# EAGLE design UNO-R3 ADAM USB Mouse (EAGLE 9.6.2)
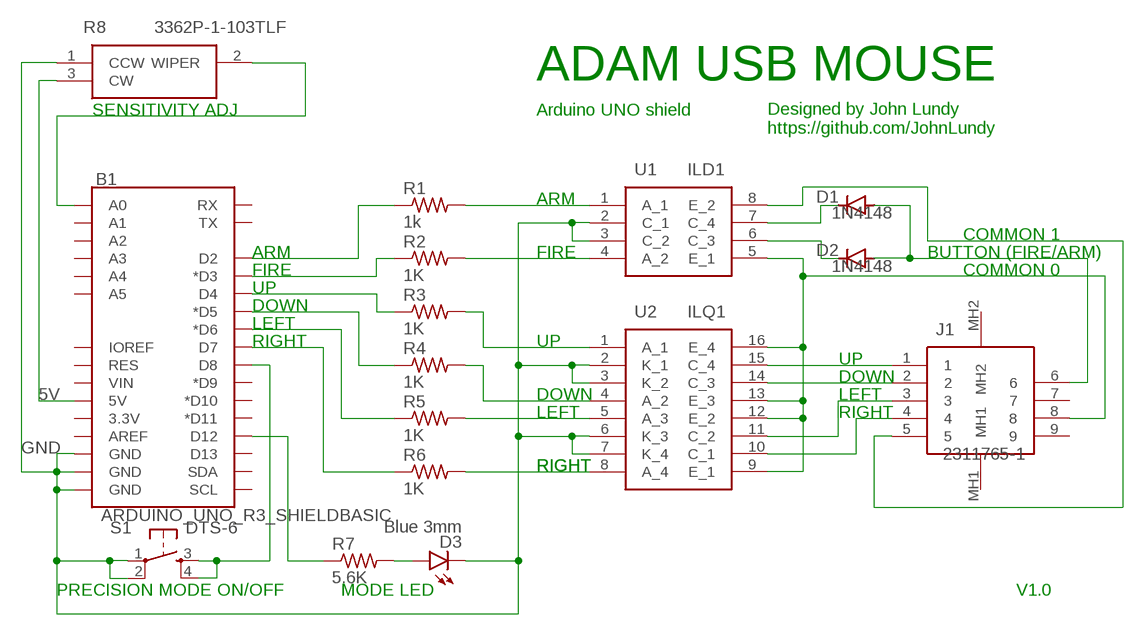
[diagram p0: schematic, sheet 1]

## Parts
B1  ARDUINO_UNO_R3_SHIELDBASIC  [UNO_R3_SHIELD]
D1  1N4148  1N4148DO35-7  [DO35-7]
D2  1N4148  1N4148DO35-7  [DO35-7]
D3  Blue 3mm  LED3MM  [LED3MM]
J1  2311765-1  [23117651]
R1  1k  R-US_0204/7  [0204/7]
R2  1K  R-US_0204/7  [0204/7]
R3  1K  R-US_0204/7  [0204/7]
R4  1K  R-US_0204/7  [0204/7]
R5  1K  R-US_0204/7  [0204/7]
R6  1K  R-US_0204/7  [0204/7]
R7  5.6K  R-US_0204/7  [0204/7]
R8  3362P-1-103TLF  [3296P-1-103]
S1  DTS-6  [DTS-6]
U1  ILD1  ILD2  [DIP762W56P254L977H470Q8N]
U2  ILQ1  [DIP762W56P254L1992H470Q16N]

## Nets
5V [Supply]: B1.5V R8.3(CW)
GND [Supply]: B1.GND@0(GND) B1.GND@1(GND) B1.GND@2(GND) D3.K(C) R8.1(CCW) S1.1 S1.2 U1.2(C_1) U1.3(C_2) U2.2(K_1) U2.3(K_2) U2.6(K_3) U2.7(K_4)
N$1: B1.D2 R1.1
N$2: B1.D3(*D3) R2.1
N$3: B1.D4 R3.1
N$4: B1.D5(*D5) R4.1
N$5: B1.D6(*D6) R5.1
N$6: B1.D7 R6.1
N$7: R1.2 U1.1(A_1)
N$8: R2.2 U1.4(A_2)
N$9: R3.2 U2.1(A_1)
N$10: R4.2 U2.4(A_2)
N$11: R5.2 U2.5(A_3)
N$12: R6.2 U2.8(A_4)
N$13: D1.C U1.7(C_4)
N$14: D2.C U1.6(C_3)
N$15: J1.5 U1.8(E_2)
N$17: J1.1 U2.15(C_4)
N$18: J1.8 U1.5(E_1) U2.9(E_1) U2.12(E_2) U2.13(E_3) U2.16(E_4)
N$20: B1.A0 R8.2(WIPER)
N$21: B1.D8 S1.3 S1.4
N$22: B1.D12 R7.1
N$23: D3.A R7.2
N$24: J1.2 U2.14(C_3)
N$25: D1.A D2.A J1.6
N$26: J1.3 U2.11(C_2)
N$27: J1.4 U2.10(C_1)
Unconnected: B1.3.3V B1.A1 B1.A2 B1.A3 B1.A4 B1.A5 B1.AREF B1.D9(*D9) B1.D10(*D10) B1.D11(*D11) B1.D13 B1.IOREF B1.RES B1.RX B1.SCL B1.SDA B1.TX B1.VIN J1.7 J1.9 J1.MH1 J1.MH2

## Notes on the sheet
- ADAM USB MOUSE
- SENSITIVITY ADJ | Arduino UNO shield
- Designed by John Lundy
  https://github.com/JohnLundy
- ARM
- COMMON 1
- ARM | FIRE | BUTTON (FIRE/ARM)
- FIRE | COMMON 0
- UP
- DOWN
- LEFT
- RIGHT | UP
- UP
- DOWN
- DOWN | LEFT
- LEFT | RIGHT
- RIGHT | RIGHT
- PRECISION MODE ON/OFF | MODE LED | V1.0

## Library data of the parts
B1 = SparkFun-Boards:ARDUINO_UNO_R3_SHIELD: Arduino R3 Shield Footprint Shield form compatible with the Arduino Uno R3. SparkFun Products: MG2639 Cellular Shield MIDI Shield R3 Stackable Headers Kit
D1 D2 = diode:1N4148: DIODE
D3 = led:LED: LED
J1 = SamacSys_Parts:2311765-1: AMPLIMITE HD22 Board Mount Connectors: AMPL REC, HD20, R/A, 9P, S/L, .318 Source: Datasheet; ARROW_PART_NUMBER: 2311765-1; ARROW_PRICE-STOCK: https://www.arrow.com/en/products/2311765-1/te-connectivity; DESCRIPTION: AMPLIMITE HD22 Board Mount Connectors: AMPL REC, HD20, R/A, 9P, S/L, .318; HEIGHT: 12.8mm; MANUFACTURER_NAME: TE Connectivity; MANUFACTURER_PART_NUMBER: 2311765-1; MOUSER_PART_NUMBER: 571-2311765-1; MOUSER_PRICE-STOCK: https://www.mouser.co.uk/ProductDetail/TE-Connectivity/2311765-1?qs=rrS6PyfT74ebQi5fQFugmA%3D%3D
R1-R7 = adafruit:R-US_: RESISTOR, American symbol
R8 = SamacSys_Parts:3362P-1-103TLF: BOURNS - 3362P-1-103TLF - TRIMMER POTENTIOMETER, 10KOHM 1TURN THROUGH HOLE Source: Datasheet; ARROW_PART_NUMBER: 3362P-1-103TLF; ARROW_PRICE-STOCK: https://www.arrow.com/en/products/3362p-1-103tlf/bourns; DESCRIPTION: BOURNS - 3362P-1-103TLF - TRIMMER POTENTIOMETER, 10KOHM 1TURN THROUGH HOLE; HEIGHT: mm; MANUFACTURER_NAME: Bourns; MANUFACTURER_PART_NUMBER: 3362P-1-103TLF; MOUSER_PART_NUMBER: 652-3362P-1-103TLF; MOUSER_PRICE-STOCK: https://www.mouser.co.uk/ProductDetail/Bourns/3362P-1-103TLF?qs=izR6mho4f8VBTlFqy0U7Gg%3D%3D
S1 = switch-tact:DTS-6
U1 = SamacSys_Parts:ILD2: Transistor Output Optocouplers Phototransistor Out Dual CTR >100% Source: Datasheet; ARROW_PART_NUMBER: ILD2; ARROW_PRICE-STOCK: https://www.arrow.com/en/products/ild2/vishay; DESCRIPTION: Transistor Output Optocouplers Phototransistor Out Dual CTR >100%; HEIGHT: 4.7mm; MANUFACTURER_NAME: Vishay; MANUFACTURER_PART_NUMBER: ILD2; MOUSER_PART_NUMBER: 782-ILD2; MOUSER_PRICE-STOCK: https://www.mouser.co.uk/ProductDetail/Vishay-Semiconductors/ILD2/?qs=xCMk%252BIHWTZN1gQU5Qacjxw%3D%3D
U2 = SamacSys_Parts:ILQ1: Optocoupler DC-IN 4-CH Trans DC-OUT Source: Datasheet; ARROW_PART_NUMBER: ILQ1; ARROW_PRICE-STOCK: https://www.arrow.com/en/products/ilq1/vishay; DESCRIPTION: Optocoupler DC-IN 4-CH Trans DC-OUT; HEIGHT: 4.7mm; MANUFACTURER_NAME: Vishay; MANUFACTURER_PART_NUMBER: ILQ1; MOUSER_PART_NUMBER: 782-ILQ1; MOUSER_PRICE-STOCK: https://www.mouser.co.uk/ProductDetail/Vishay-Semiconductors/ILQ1?qs=MZ2FkKEZZL8rYKp%252BhEUQuQ%3D%3D

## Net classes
0 default: width 0.3 mm
1 Supply: width 0.5 mm

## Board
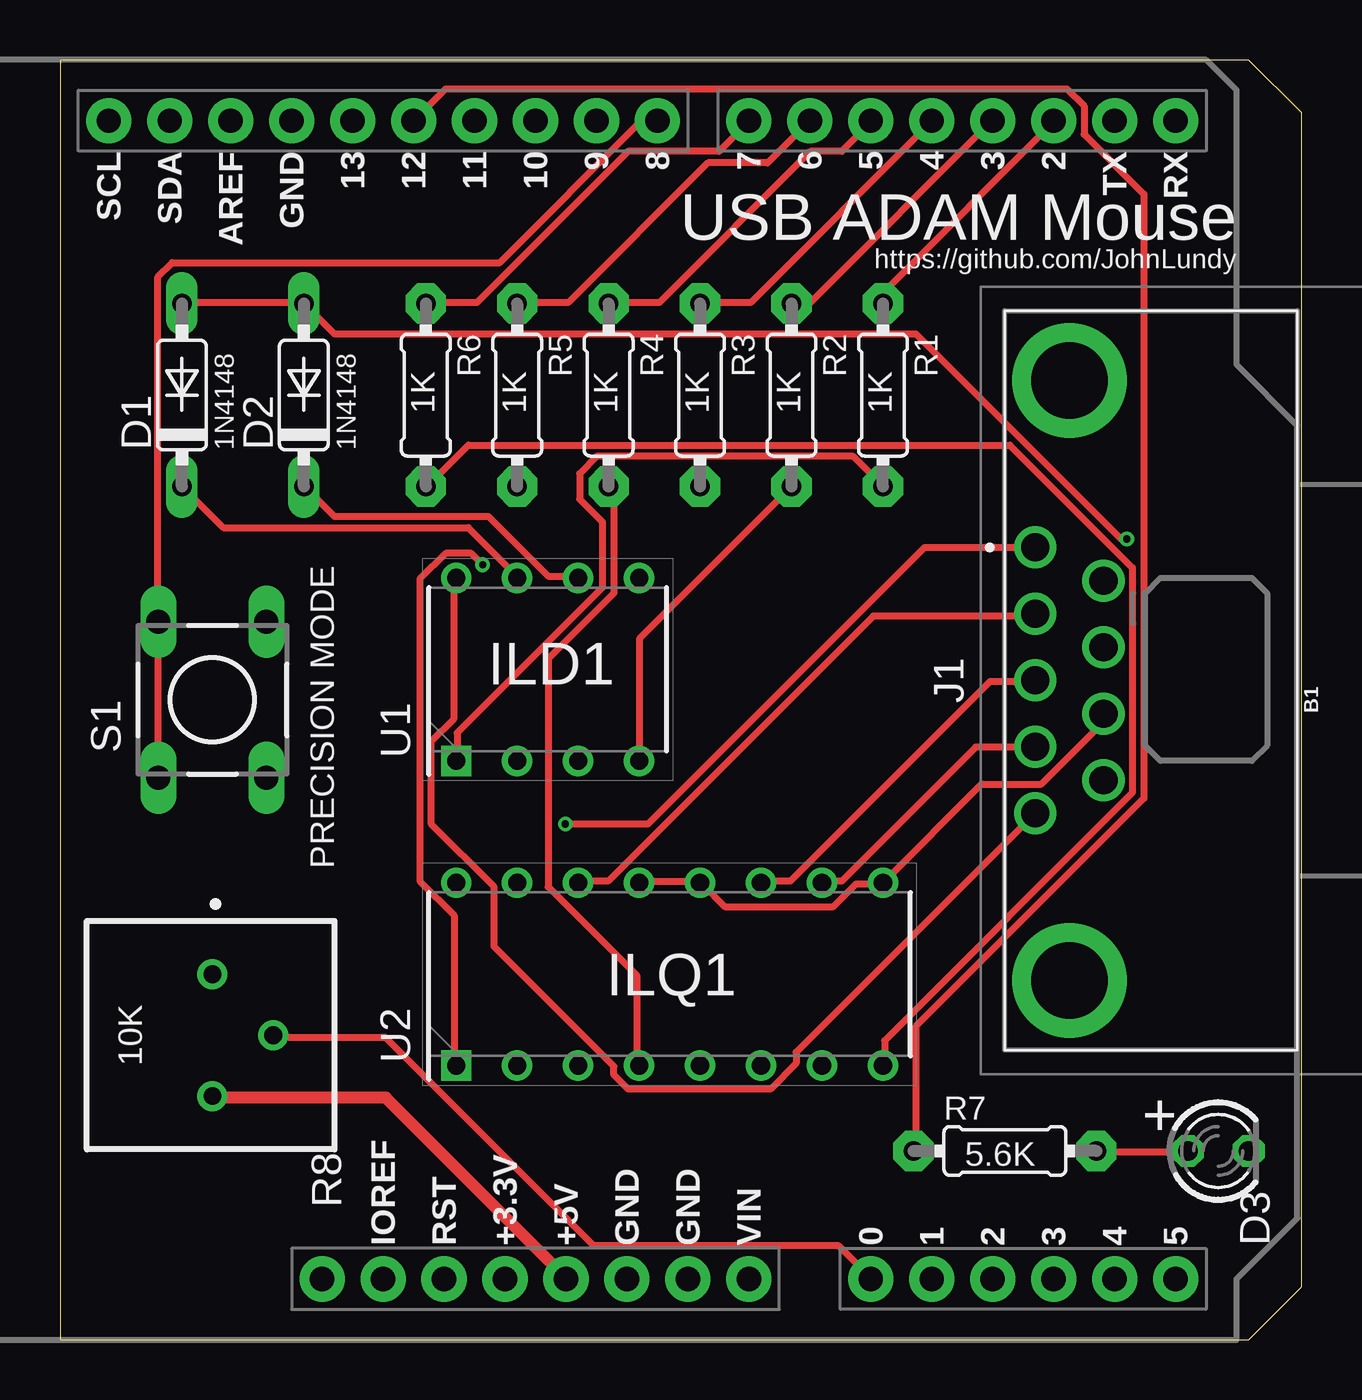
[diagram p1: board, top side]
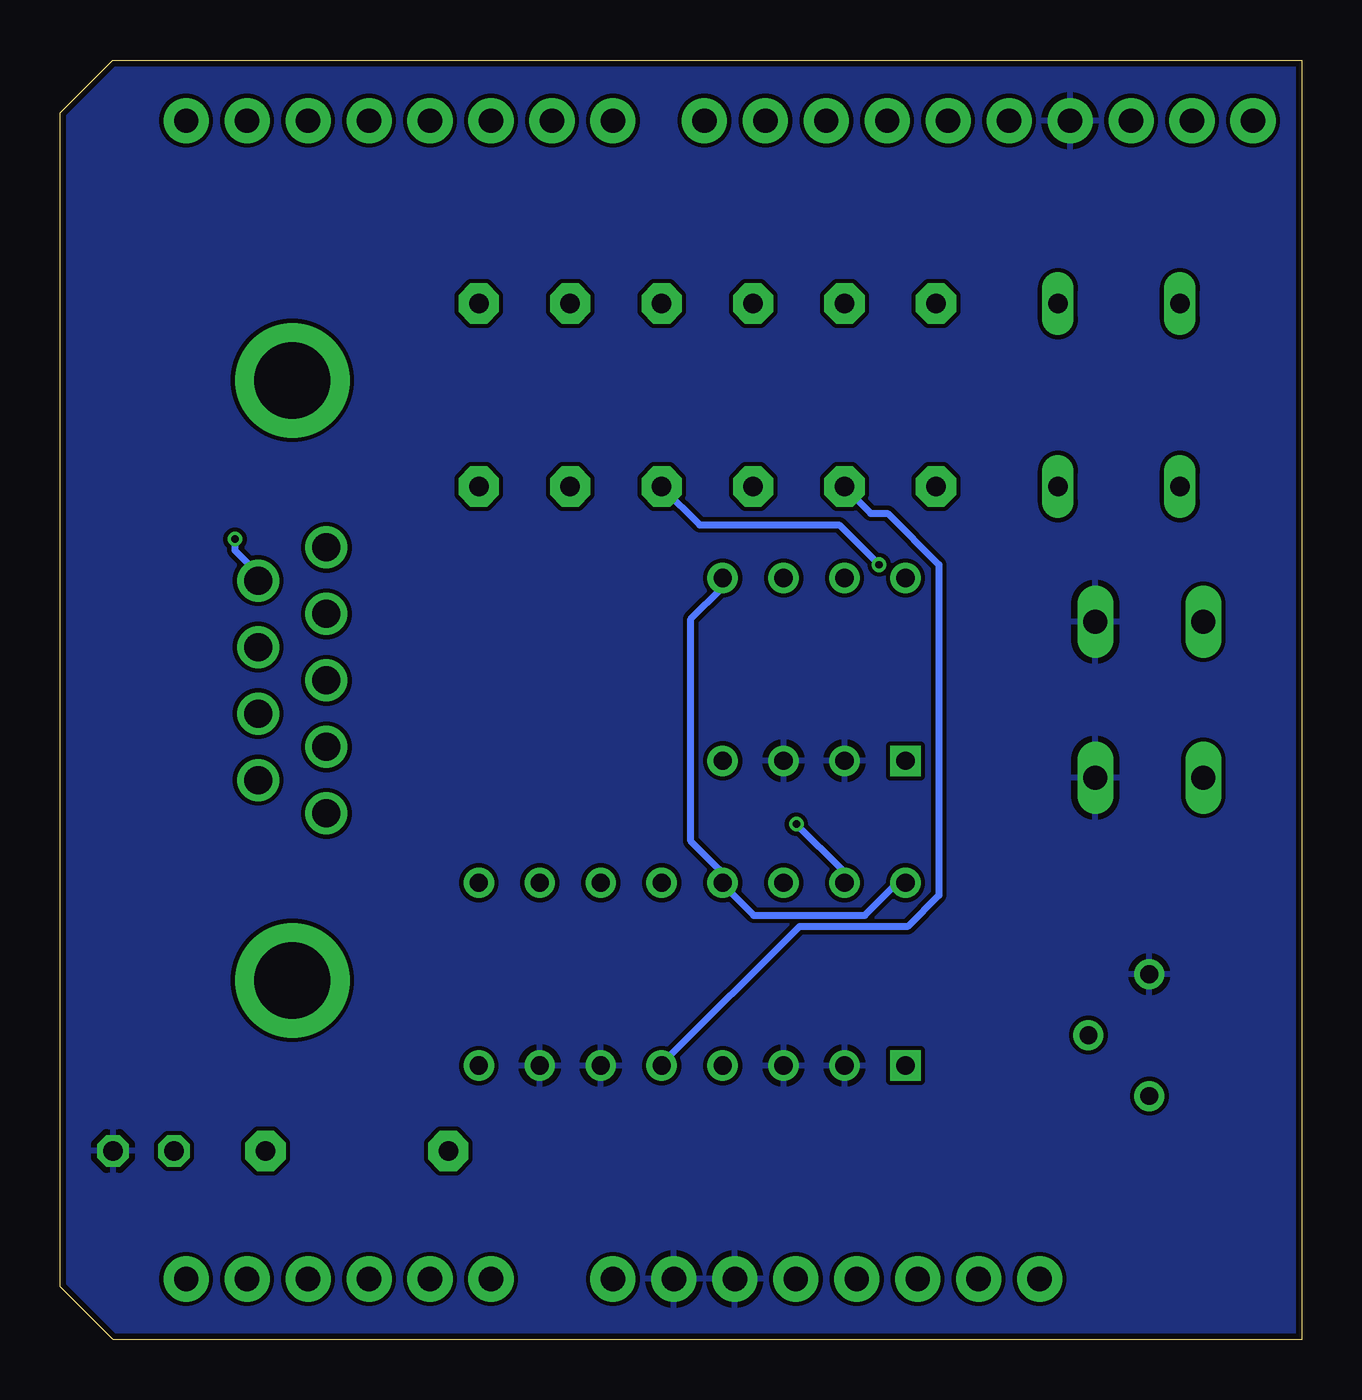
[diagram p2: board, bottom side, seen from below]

Size 51.74 x 53.33 mm. Coordinates in mm from the lower left corner, seen from the top.
Outline: 0,0 49.53,0 51.74,2.21 51.74,51.13 49.54,53.33 0,53.33 0,0
Copper layers (1*16): Top 0.035mm / dielectric 1.5mm / Bottom 0.035mm
Design rules "dirt_cheap_dirty_boards.v1.1 *": minimum track width 6mil, minimum drill 12mil, track to track 0.175mm, track to pad 0.175mm, pad to pad 0.175mm, via to via 6mil, smd to smd 0mil, copper to edge 10mil, drill to drill 10mil, minimum pad ring 10mil, minimum via ring 6mil, stop-mask expansion 2mil, vias tented up to drill 25mil, thermal gap 10mil

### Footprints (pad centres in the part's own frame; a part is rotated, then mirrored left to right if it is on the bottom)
UNO_R3_SHIELD = drill 1.016 pad 1.88: 3.3V 24.13,-2.54; 5V 24.13,0; A0 24.13,12.7; A1 24.13,15.24; A2 24.13,17.78; A3 24.13,20.32; A4 24.13,22.86; A5 24.13,25.4; AREF -24.13,-13.97; D2 -24.13,20.32; D3 -24.13,17.78; D4 -24.13,15.24; D5 -24.13,12.7; D6 -24.13,10.16; D7 -24.13,7.62; D8 -24.13,3.81; D9 -24.13,1.27; D10 -24.13,-1.27; D11 -24.13,-3.81; D12 -24.13,-6.35; D13 -24.13,-8.89; GND@0 24.13,2.54; GND@1 24.13,5.08; GND@2 -24.13,-11.43; IOREF 24.13,-7.62; NC 24.13,-10.16; RES 24.13,-5.08; RX -24.13,25.4; SCL -24.13,-19.05; SDA -24.13,-16.51; TX -24.13,22.86; VIN 24.13,7.62
DO35-7 = drill 0.813 long: A 3.81,0; C -3.81,0
LED3MM = drill 0.813 octagon: A -1.27,0; K 1.27,0
23117651 = drill 1.17 pad 1.755: 1 0,0; 2 -2.77,0; 3 -5.54,0; 4 -8.31,0; 5 -11.08,0; 6 -1.385,-2.84; 7 -4.155,-2.84; 8 -6.925,-2.84; 9 -9.695,-2.84 | drill 3.18 pad 4.77: MH1 -18.04,-1.42; MH2 6.96,-1.42
0204/7 = drill 0.813 pad 1.676 octagon: 1 -3.81,0; 2 3.81,0
3296P-1-103 = drill 0.74 pad 1.24: 1 -2.54,-2.54; 2 0,0; 3 2.54,-2.54
DTS-6 = drill 1 long: 1 -3.25,2.25; 2 3.25,2.25; 3 -3.25,-2.25; 4 3.25,-2.25
DIP762W56P254L977H470Q8N = drill 0.76 pad 1.16 square: 1 -3.81,3.81 | drill 0.76 pad 1.16: 2 -3.81,1.27; 3 -3.81,-1.27; 4 -3.81,-3.81; 5 3.81,-3.81; 6 3.81,-1.27; 7 3.81,1.27; 8 3.81,3.81
DIP762W56P254L1992H470Q16N = drill 0.76 pad 1.16 square: 1 -3.81,8.89 | drill 0.76 pad 1.16: 2 -3.81,6.35; 3 -3.81,3.81; 4 -3.81,1.27; 5 -3.81,-1.27; 6 -3.81,-3.81; 7 -3.81,-6.35; 8 -3.81,-8.89; 9 3.81,-8.89; 10 3.81,-6.35; 11 3.81,-3.81; 12 3.81,-1.27; 13 3.81,1.27; 14 3.81,3.81; 15 3.81,6.35; 16 3.81,8.89

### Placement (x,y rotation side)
B1  21.08,26.67 270 top
D1  5.08,39.37 90 top
D2  10.16,39.37 90 top
D3  48.26,7.87 0 top
J1  40.64,33.02 90 top
R1  34.29,39.37 270 top
R2  30.48,39.37 270 top
R3  26.67,39.37 270 top
R4  22.86,39.37 270 top
R5  19.05,39.37 270 top
R6  15.24,39.37 270 top
R7  39.37,7.87 0 top
R8  8.89,12.7 270 top
S1  6.35,26.67 270 top
U1  20.32,27.94 90 top
U2  25.4,15.24 90 top

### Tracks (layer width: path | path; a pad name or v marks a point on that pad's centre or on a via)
5V
  Top 0.5: R8.3 6.45,10.09 13.57,10.09 21.05,2.61 B1.5V
GND
  pour Bottom: 0,53.34 49.53,53.34 52.07,50.8 52.07,2.54 49.53,0 0,0
N$1
  Top 0.3: R1.1 34.35,43.23 34.35,43.7 41.36,50.71 B1.D2
N$2
  Top 0.3: R2.1 30.55,43.23 31.27,43.23 38.75,50.71 B1.D3
N$3
  Top 0.3: R3.1 26.75,43.23 28.77,43.23 36.25,50.71 B1.D4
N$4
  Top 0.3: R4.1 22.96,43.23 24.97,43.23 31.27,49.52 32.57,49.52 33.76,50.71 B1.D5
N$5
  Top 0.3: R5.1 19.16,43.23 21.17,43.23 26.99,49.04 29.49,49.04 31.15,50.71 B1.D6
N$6
  Top 0.3: R6.1 15.36,43.23 17.37,43.23 23.67,49.52 27.47,49.52 28.66,50.71 B1.D7
N$7
  Top 0.3: U1.1 16.54,24.23 16.54,25.29 22.6,31.35 22.6,34.08 21.65,35.03 21.65,36.1 22.36,36.81 33.05,36.81 34.24,35.62 R1.2
N$8
  Top 0.3: U1.4 24.14,24.23 24.14,29.21 30.44,35.51 R2.2
N$9  (via drill 0.3)
  Top 0.3: v17.61,32.3 17.14,32.77 16.07,32.77 15,31.71 15,19.12 16.42,17.69 16.42,11.52 U2.1
  Bottom 0.3: v17.61,32.3 19.27,33.96 25.09,33.96 26.64,35.51 R3.2
N$10
  Top 0.3: U2.4 24.02,11.52 24.02,15.2 20.34,18.88 20.34,28.38 23.07,31.11 23.07,35.39 22.96,35.51 R4.2
N$11
  Bottom 0.3: U2.5 26.64,11.52 20.94,17.22 16.42,17.22 15.12,18.52 15.12,32.3 17.25,34.44 17.97,34.44 19.04,35.51 R5.2
N$12
  Top 0.3: U2.8 34.35,11.52 34.35,12.47 44.69,22.8 44.69,32.18 39.58,37.29 17.02,37.29 15.36,35.62 R6.2
N$13
  Top 0.3: U1.7 19.04,31.82 17.02,33.84 6.8,33.84 5.14,35.51 D1.C
N$14
  Top 0.3: U1.6 21.53,31.82 20.34,31.82 17.85,34.32 11.44,34.32 10.25,35.51 D2.C
N$15
  Top 0.3: U1.8 16.42,31.71 16.42,25.89 15.47,24.94 15.47,21.49 18.09,18.88 18.09,16.39 23.07,11.4 23.07,11.04 23.67,10.45 29.61,10.45 30.67,11.52 30.67,11.99 40.53,21.85 J1.5
N$17  (via drill 0.3)
  Top 0.3: v21.05,21.49 24.5,21.49 36.02,33.01 40.53,33.01 J1.1
  Bottom 0.3: v21.05,21.49 19.16,19.59 19.16,19.12 U2.15
N$18
  Top 0.3: U2.13 24.14,19.12 26.64,19.12 U2.12 26.75,19 27.71,18.05 32.22,18.05 33.17,19 34.24,19 U2.9 34.35,19.12 38.39,23.16 40.89,23.16 43.38,25.65 43.38,26.01 J1.8
  Bottom 0.3: U2.16 16.54,19 16.9,19 18.21,17.69 22.84,17.69 24.14,19 U2.13 24.26,19.12 24.26,19.59 25.45,20.78 25.45,30.04 24.14,31.35 24.14,31.71 U1.5
N$20
  Top 0.3: R8.2 8.94,12.59 13.57,12.59 22.24,3.92 32.45,3.92 33.76,2.61 B1.A0
N$21
  Top 0.3: S1.4 4.07,23.51 4.07,29.81 S1.3 4.07,30.04 4.07,44.29 4.67,44.89 18.32,44.89 24.14,50.71 24.86,50.71 B1.D8
N$22
  Top 0.3: R7.1 35.66,7.96 35.66,13.06 45.16,22.56 45.16,47.74 42.67,50.23 42.67,51.42 41.95,52.13 16.07,52.13 14.76,50.83 B1.D12
N$23
  Top 0.3: D3.A 46.94,7.84 43.26,7.84 R7.2
N$24
  Top 0.3: U2.14 21.65,19.12 22.84,19.12 33.88,30.16 40.53,30.16 J1.2
N$25  (via drill 0.3)
  Top 0.3: D1.A 5.14,43.23 10.13,43.23 D2.A 10.25,43.11 11.44,41.92 35.66,41.92 44.21,33.37 v44.45,33.37
  Bottom 0.3: v44.45,33.37 44.45,32.89 43.5,31.94 43.5,31.71 J1.6
N$26
  Top 0.3: U2.11 29.25,19.12 30.44,19.12 38.75,27.43 40.53,27.43 J1.3
N$27
  Top 0.3: U2.10 31.86,19.12 32.57,19.12 38.15,24.7 40.53,24.7 J1.4

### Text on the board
tNames: USB ADAM Mouse | https://github.com/JohnLundy | 1K | 1K | 1K | 1K | 1K | 1K | 1N4148 | 1N4148 | PRECISION MODE | ILD1 | ILQ1 | 10K | + | 5.6K

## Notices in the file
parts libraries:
SparkFun-Boards: Licensing: Creative Commons ShareAlike 4.0 International - https://creativecommons.org/licenses/by-sa/4.0
